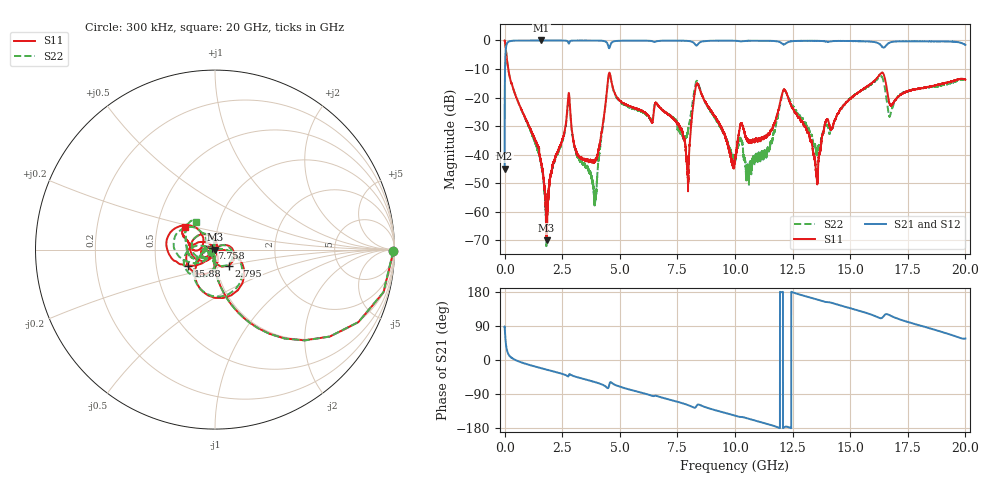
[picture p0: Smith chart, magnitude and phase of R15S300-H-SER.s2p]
!{R15S300}
!Johanson Technology Inc.
!www.johansontechnology.com
!Test Board Conditions:
!Substrate Type  RO4350B
!Substrate Thickness  20 mil
!Substrate Dk  3.66
!TL Type: GCPW
!TL Trace Width  34 mil
!TL Gap  10 mil
!Electrode orientation  Horizontal
!DUT TOPOLOGY	SERIES
!Mounting Pad LxW  26x52 mil
! Created Sat Feb  6 14:25:15 2021
# hz S ma R 50
! 2 Port Network Data from SP1.SP block
! freq  magS11  angS11  magS21  angS21  magS12  angS12  magS22  angS22
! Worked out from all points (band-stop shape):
!   20001 points, 300 kHz to 20 GHz, reference 50 ohm
!   highest |S21| = 0.00 dB at 1.596 GHz (marker M1); lowest = -44.9 dB at 300 kHz (marker M2)
!   |S21| within 3 dB of the highest: 53.4 MHz to end of sweep
!   lowest |S11| = -70.0 dB at 1.822 GHz (marker M3), VSWR 1.00, Z = 50 - j0.00661 ohm
!   |S11| at or under -10 dB: 157.9 MHz to end of sweep
!   |S22| runs from -72.0 to 0.0 dB; largest |S21 - S12| = 0.013
!   S11 on the Smith chart (normalised r, x): 300 kHz: open; 2.795 GHz: 1.15, -0.21; 7.758 GHz: 0.96, +0.02; 15.88 GHz: 0.73, -0.14; 20 GHz: 0.70, +0.19
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300000  0.9944 -0.5  0.005667 88.2  0.005607 90.4  0.9932 -0.4
1.493e8  0.3324 -72.5  0.9405 17.4  0.9411 17.2  0.3343 -72.5
1.5963e9  0.006877 -111.7  0.9999 -21.8  0.9987 -21.8  0.006547 -108.4
1.8223e9  0.0003177 -12.0  0.9986 -25.4  0.9985 -25.4  0.0004639 -4.0
2.7953e9  0.1182 -49.1  0.8852 -38.9  0.885 -38.9  0.1104 -52.3
3.3343e9  0.008876 -94.3  0.9959 -48.4  0.996 -48.4  0.007729 -157.3
3.9363e9  0.007882 -50.8  0.9935 -58.5  0.9941 -58.6  0.001623 89.1
4.5583e9  0.2715 -86.7  0.7487 -61.6  0.7495 -61.6  0.2618 -89.5
6.6673e9  0.0724 -179.3  0.9819 -96.1  0.9806 -96.1  0.07286 -177.4
7.7583e9  0.02104 151.1  0.9882 -114.9  0.9874 -114.8  0.01956 -160.3
7.9653e9  0.004031 -126.2  0.9792 -119.1  0.9799 -119.0  0.02772 -108.4
8.3663e9  0.1743 -151.3  0.8325 -118.6  0.8334 -118.5  0.1938 -151.7
1.00003e10  0.008363 -129.8  0.9864 -146.7  0.9865 -146.7  0.008272 -130.4
1.02763e10  0.03498 -141.2  0.9631 -150.4  0.9636 -150.4  0.01735 -176.5
1.14133e10  0.0223 -113.5  0.9862 -168.9  0.9859 -168.8  0.0127 -68.0
1.21413e10  0.1385 169.2  0.855 -177.4  0.8547 -177.6  0.1332 162.4
1.33343e10  0.0165 57.8  0.9848 163.6  0.9839 163.6  0.02157 105.6
1.35573e10  0.003496 -21.7  0.984 159.7  0.9836 159.7  0.01007 143.7
1.39613e10  0.04005 -137.9  0.9569 153.0  0.9582 152.8  0.03236 -165.6
1.58813e10  0.1734 -148.5  0.9553 120.5  0.9555 120.6  0.168 -156.3
1.66673e10  0.09186 135.5  0.897 119.5  0.891 119.8  0.053 149.5
2e10  0.2067 141.8  0.8412 56.8  0.8391 56.7  0.1858 124.3
